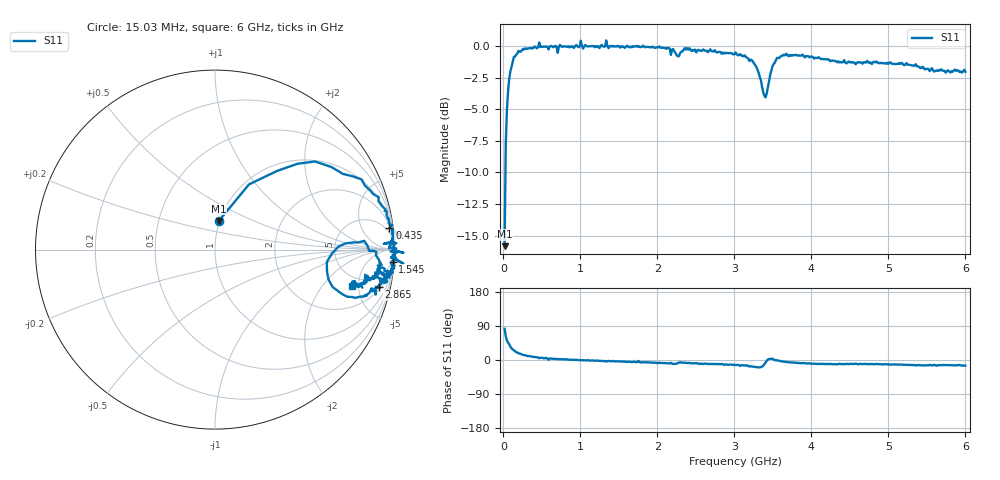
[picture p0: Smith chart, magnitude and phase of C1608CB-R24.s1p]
!	Network	Analyzer	HP8753E.07.74:	Oct	30	2002	Serial	No.	JP38451487
!	Hewlett-Packard
!	28	Aug	2009	8:30:54
!	Frequency	S11
#	HZ	S	RI	R	50
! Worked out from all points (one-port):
!   400 points, 15.03 MHz to 6 GHz, reference 50 ohm
!   lowest |S11| = -15.8 dB at 15.03 MHz (marker M1), VSWR 1.39, Z = 49.6 + j16.3 ohm
!   |S11| at or under -10 dB: start of sweep to 25.87 MHz
!   S11 on the Smith chart (normalised r, x): 15.03 MHz: 0.99, +0.33; 435 MHz: 3, +16; 1.545 GHz: 3, -29; 2.865 GHz: 2.45, -8.10; 6 GHz: 3.89, -4.21
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1.502992e7  0.0217 0.16
3.002985e7  0.189 0.363
6.00297e7  0.459 0.478
9.002955e7  0.649 0.46
1.95029e8  0.912 0.292
4.350278e8  0.972 0.122
5.550272e8  0.992 0.0973
5.850271e8  0.97 0.00714
7.650262e8  0.992 0.0446
1.005025e9  1.05 -0.0172
1.035025e9  0.978 -0.00946
1.245024e9  0.981 -0.0439
1.335023e9  1.05 -0.0782
1.365023e9  0.981 -0.0427
1.515022e9  0.984 -0.0659
1.545022e9  0.99 -0.0664
2.265019e9  0.902 -0.131
2.355018e9  0.974 -0.124
2.865016e9  0.911 -0.209
3.015015e9  0.919 -0.215
3.315013e9  0.738 -0.263
3.405013e9  0.623 -0.0691
3.465013e9  0.77 0.0401
3.555012e9  0.899 -0.0135
3.765011e9  0.913 -0.104
4.515007e9  0.852 -0.152
5.265004e9  0.822 -0.19
6e9  0.765 -0.202
